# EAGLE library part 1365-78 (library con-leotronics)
DUAL ROW STRAIGHT HEADER 1364 SERIES. 1.27mm x 1.27mm. Without Fixing Post. SMT Source: http://www.leotronics.co.uk/Conexcon/Data%20Sheets/sec.%20A/1364ing.pdf
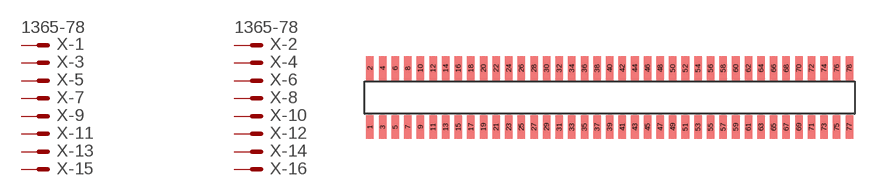
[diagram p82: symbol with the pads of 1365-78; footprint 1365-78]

Designator prefix X; gates -1=MVAL -2=MVAL -3=M -4=M -5=M -6=M -7=M -8=M -9=M -10=M -11=M -12=M -13=M -14=M -15=M -16=M -17=M -18=M -19=M -20=M -21=M -22=M -23=M -24=M -25=M -26=M -27=M -28=M -29=M -30=M -31=M -32=M -33=M -34=M -35=M -36=M -37=M -38=M -39=M -40=M -41=M -42=M -43=M -44=M -45=M -46=M -47=M -48=M -49=M -50=M -51=M -52=M -53=M -54=M -55=M -56=M -57=M -58=M -59=M -60=M -61=M -62=M -63=M -64=M -65=M -66=M -67=M -68=M -69=M -70=M -71=M -72=M -73=M -74=M -75=M -76=M -77=M -78=M

## 1365-78 (OC_FARNELL: unknown; OC_NEWARK: unknown)  [1365-78]
1  -1:S  pas
2  -2:S  pas
3  -3:S  pas
4  -4:S  pas
5  -5:S  pas
6  -6:S  pas
7  -7:S  pas
8  -8:S  pas
9  -9:S  pas
10  -10:S  pas
11  -11:S  pas
12  -12:S  pas
13  -13:S  pas
14  -14:S  pas
15  -15:S  pas
16  -16:S  pas
17  -17:S  pas
18  -18:S  pas
19  -19:S  pas
20  -20:S  pas
21  -21:S  pas
22  -22:S  pas
23  -23:S  pas
24  -24:S  pas
25  -25:S  pas
26  -26:S  pas
27  -27:S  pas
28  -28:S  pas
29  -29:S  pas
30  -30:S  pas
31  -31:S  pas
32  -32:S  pas
33  -33:S  pas
34  -34:S  pas
35  -35:S  pas
36  -36:S  pas
37  -37:S  pas
38  -38:S  pas
39  -39:S  pas
40  -40:S  pas
41  -41:S  pas
42  -42:S  pas
43  -43:S  pas
44  -44:S  pas
45  -45:S  pas
46  -46:S  pas
47  -47:S  pas
48  -48:S  pas
49  -49:S  pas
50  -50:S  pas
51  -51:S  pas
52  -52:S  pas
53  -53:S  pas
54  -54:S  pas
55  -55:S  pas
56  -56:S  pas
57  -57:S  pas
58  -58:S  pas
59  -59:S  pas
60  -60:S  pas
61  -61:S  pas
62  -62:S  pas
63  -63:S  pas
64  -64:S  pas
65  -65:S  pas
66  -66:S  pas
67  -67:S  pas
68  -68:S  pas
69  -69:S  pas
70  -70:S  pas
71  -71:S  pas
72  -72:S  pas
73  -73:S  pas
74  -74:S  pas
75  -75:S  pas
76  -76:S  pas
77  -77:S  pas
78  -78:S  pas

## Footprint 1365-78 (pad centres in mm)
DUAL ROW STRAIGHT HEADER 1364 SERIES. 1.27mm x 1.27mm. Without Fixing Post. SMT Source: http://www.leotronics.co.uk/Conexcon/Data%20Sheets/sec.%20A/1364ing.pdf
smd 0.76 x 2.4: 1 -24.13,-2.95; 2 -24.13,2.95; 3 -22.86,-2.95; 4 -22.86,2.95; 5 -21.59,-2.95; 6 -21.59,2.95; 7 -20.32,-2.95; 8 -20.32,2.95; 9 -19.05,-2.95; 10 -19.05,2.95; 11 -17.78,-2.95; 12 -17.78,2.95; 13 -16.51,-2.95; 14 -16.51,2.95; 15 -15.24,-2.95; 16 -15.24,2.95; 17 -13.97,-2.95; 18 -13.97,2.95; 19 -12.7,-2.95; 20 -12.7,2.95; 21 -11.43,-2.95; 22 -11.43,2.95; 23 -10.16,-2.95; 24 -10.16,2.95; 25 -8.89,-2.95; 26 -8.89,2.95; 27 -7.62,-2.95; 28 -7.62,2.95; 29 -6.35,-2.95; 30 -6.35,2.95; 31 -5.08,-2.95; 32 -5.08,2.95; 33 -3.81,-2.95; 34 -3.81,2.95; 35 -2.54,-2.95; 36 -2.54,2.95; 37 -1.27,-2.95; 38 -1.27,2.95; 39 0,-2.95; 40 0,2.95; 41 1.27,-2.95; 42 1.27,2.95; 43 2.54,-2.95; 44 2.54,2.95; 45 3.81,-2.95; 46 3.81,2.95; 47 5.08,-2.95; 48 5.08,2.95; 49 6.35,-2.95; 50 6.35,2.95; 51 7.62,-2.95; 52 7.62,2.95; 53 8.89,-2.95; 54 8.89,2.95; 55 10.16,-2.95; 56 10.16,2.95; 57 11.43,-2.95; 58 11.43,2.95; 59 12.7,-2.95; 60 12.7,2.95; 61 13.97,-2.95; 62 13.97,2.95; 63 15.24,-2.95; 64 15.24,2.95; 65 16.51,-2.95; 66 16.51,2.95; 67 17.78,-2.95; 68 17.78,2.95; 69 19.05,-2.95; 70 19.05,2.95; 71 20.32,-2.95; 72 20.32,2.95; 73 21.59,-2.95; 74 21.59,2.95; 75 22.86,-2.95; 76 22.86,2.95; 77 24.13,-2.95; 78 24.13,2.95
